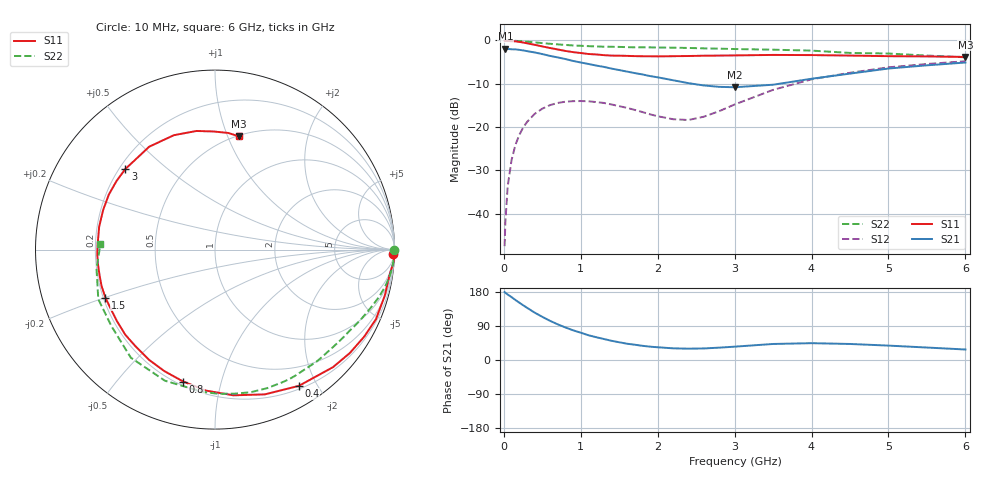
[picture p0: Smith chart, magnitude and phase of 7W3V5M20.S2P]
! Infineon Technologies  Discrete & RF Semiconductors
! BFS17W
! Si NPN RF Bipolar Junction Transistor in SOT323
! VCE = 3.5 V  IC = 0.2 mA
! Common Emitter S-Parameters:  August  1999
# GHz  S  MA  R  50
!  f  S11  S21  S12  S22
! GHz  MAG  ANG  MAG  ANG  MAG  ANG  MAG  ANG
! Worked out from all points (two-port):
!   36 points, 10 MHz to 6 GHz, reference 50 ohm
!   highest |S21| = -1.91 dB at 20 MHz (marker M1); lowest = -10.8 dB at 3 GHz (marker M2)
!   |S21| within 3 dB of the highest: start of sweep to 947.5 MHz
!   lowest |S11| = -3.8 dB at 6 GHz (marker M3), VSWR 4.64, Z = 25.3 + j54.8 ohm
!   |S11| at or under -10 dB: nowhere
!   |S22| runs from -3.9 to 0.0 dB; largest |S21 - S12| = 0.8
!   S11 on the Smith chart (normalised r, x): 10 MHz: 29, -70; 400 MHz: 0.24, -1.76; 800 MHz: 0.22, -0.76; 1.5 GHz: 0.21, -0.20; 3 GHz: 0.22, +0.37; 6 GHz: 0.51, +1.10
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0.01  0.9899 -1.4  0.797 179.4  0.0042 81.7  0.9999 0.0
0.02  0.9999 -3.4  0.803 177.3  0.008 87.9  0.9973 -0.9
0.05  0.9838 -7.7  0.798 172.8  0.0206 85.6  0.9978 -2.2
0.1  0.9802 -15.1  0.791 166.0  0.0414 81.0  0.9953 -4.4
0.15  0.977 -23.4  0.789 158.5  0.0619 75.0  0.9898 -6.6
0.25  0.9468 -37.5  0.768 144.6  0.098 66.2  0.9763 -10.6
0.4  0.8914 -58.4  0.727 125.1  0.1417 53.8  0.9505 -16.2
0.6  0.8183 -82.8  0.663 103.4  0.179 40.2  0.9151 -22.6
0.8  0.7563 -103.5  0.61 85.9  0.1961 30.2  0.8874 -28.5
1.1  0.6974 -129.4  0.535 65.3  0.1983 18.9  0.8596 -36.7
1.5  0.6667 -156.3  0.455 46.8  0.1742 11.7  0.8423 -48.0
1.8  0.6571 -172.9  0.405 37.5  0.149 12.4  0.8328 -57.2
2.2  0.6579 168.8  0.347 30.8  0.123 26.5  0.8248 -69.4
2.4  0.6611 160.5  0.321 29.9  0.1205 38.2  0.8193 -75.9
2.6  0.6663 152.6  0.302 30.5  0.1315 50.1  0.81 -82.3
3  0.6717 138.1  0.288 35.2  0.182 63.2  0.796 -94.8
3.5  0.6805 122.6  0.308 42.3  0.2687 64.9  0.782 -110.9
4  0.6774 109.8  0.361 44.4  0.3554 59.2  0.7632 -127.9
4.5  0.669 98.9  0.414 42.3  0.4234 51.8  0.7177 -143.5
5  0.6581 90.6  0.474 38.0  0.4892 44.4  0.7064 -157.0
5.5  0.654 83.6  0.516 32.9  0.5347 37.3  0.6687 -170.8
6  0.6454 78.2  0.556 27.7  0.5752 30.8  0.6391 177.2
